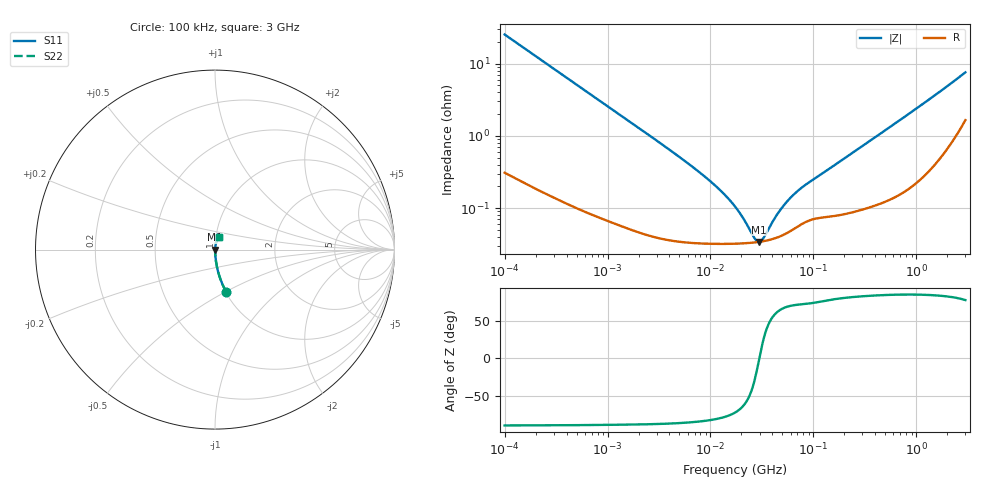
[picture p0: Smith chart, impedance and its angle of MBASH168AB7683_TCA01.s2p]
! MBASH168AB7683_TCA01  S-PARAMETER MODEL  ( Standard Model )
! Model Generated by TAIYO YUDEN Corporation (http://www.ty-top.com)
! Version 1.0
! TAIYO YUDEN Control No. 220601
! Copyright(c) 2019 TAIYO YUDEN CO.,LTD. All Rights Reserved.
! Product Description (link to TY-COMPAS)
! https://ds.yuden.co.jp/TYCOMPAS/or/detail?pn=MBASH168AB7683KTCA01&u=M
! Products Name : Multilayer Ceramic Capacitors
! Characteristics :
!  Capacitance : 0.068 [uF] , Rated Voltage : 100 [V] , TCC : X7R
!  Case Size : 1.6 x 0.8 / 0.063 x 0.031 [mm/inch] , Thickness : 0.8 / 0.031 [mm/inch]
!  (Conditions: Temperature = 25 [degC] , DC Bias Voltage = 0 [V])
! External Node Assignments :
!  1  o---| |---o  2
! GND o---------o GND
! Frequency Range : 100kHz  -  3GHz  [ 401 STEP ]
# MHZ S RI R 50
! Freq[MHz].  S11 Real  S11 Imag  S21 Real  S21 Imag  S12 Real  S12 Imag  S22 Real  S22 Imag
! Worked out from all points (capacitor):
!   401 points, 100 kHz to 3 GHz, reference 50 ohm
!   read as one part in series: C = 62.9 nF near 105.3 kHz
!   lowest |Z| = 34.1 mohm at 29.76 MHz (marker M1)
!   series resonance near 29.85 MHz, so ESL is about 450 pH
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0.1  0.0625 -0.236  0.9375 0.236  0.9375 0.236  0.0625 -0.236
0.151038  0.0294 -0.1624  0.9706 0.1624  0.9706 0.1624  0.0294 -0.1624
0.222319  0.0145 -0.1124  0.9855 0.1124  0.9855 0.1124  0.0145 -0.1124
0.562235  0.00299 -0.0454  0.997 0.0454  0.997 0.0454  0.00299 -0.0454
3.161081  0.000449 -0.00814  0.9996 0.00814  0.9996 0.00814  0.000449 -0.00814
6.178009  0.000348 -0.00404  0.9997 0.00404  0.9997 0.00404  0.000348 -0.00404
9.824692  0.000326 -0.00237  0.9997 0.00237  0.9997 0.00237  0.000326 -0.00237
13.7349  0.000321 -0.0015  0.9997 0.0015  0.9997 0.0015  0.000321 -0.0015
17.7727  0.000322 -0.00095  0.9997 0.00095  0.9997 0.00095  0.000322 -0.00095
20.74485  0.000325 -0.000652  0.9997 0.000652  0.9997 0.000652  0.000325 -0.000652
26.84345  0.000334 -0.000187  0.9997 0.000187  0.9997 0.000187  0.000334 -0.000187
28.26337  0.000337 -9.61e-05  0.9997 9.61e-05  0.9997 9.61e-05  0.000337 -9.61e-05
29.75839  0.000341 -5.61e-06  0.9997 5.61e-06  0.9997 5.61e-06  0.000341 -5.61e-06
31.3325  0.000345 8.49e-05  0.9997 -8.49e-05  0.9997 -8.49e-05  0.000345 8.49e-05
32.98988  0.000349 0.000176  0.9997 -0.000176  0.9997 -0.000176  0.000349 0.000176
43.80277  0.000388 0.000688  0.9996 -0.000688  0.9996 -0.000688  0.000388 0.000688
55.23785  0.000451 0.00114  0.9995 -0.00114  0.9995 -0.00114  0.000451 0.00114
71.47675  0.000565 0.00166  0.9994 -0.00166  0.9994 -0.00166  0.000565 0.00166
97.38194  0.000699 0.00232  0.9993 -0.00232  0.9993 -0.00232  0.000699 0.00232
547.5153  0.00146 0.013  0.9985 -0.013  0.9985 -0.013  0.00146 0.013
1420.79  0.00471 0.0336  0.9953 -0.0336  0.9953 -0.0336  0.00471 0.0336
3000  0.0214 0.071  0.9786 -0.071  0.9786 -0.071  0.0214 0.071
